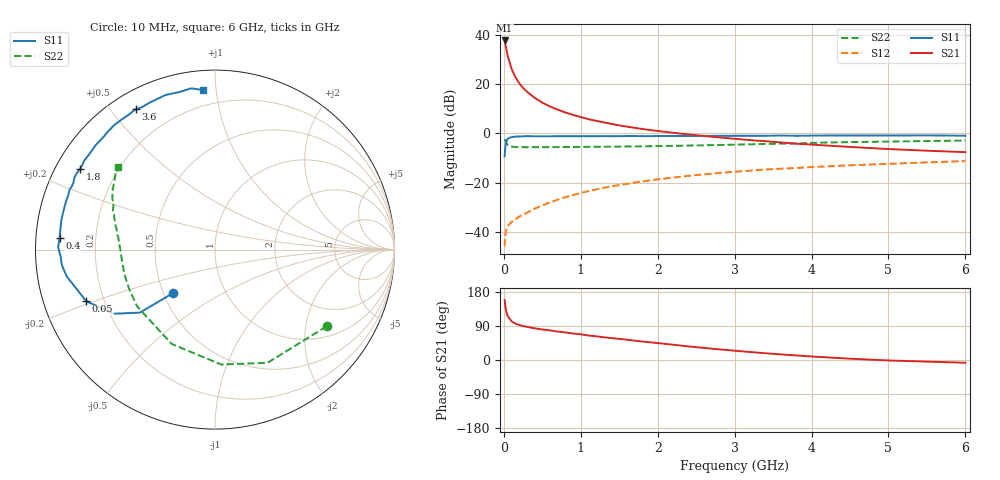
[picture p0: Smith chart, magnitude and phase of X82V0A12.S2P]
! SIEMENS Small Signal Semiconductors
! BFP136W
! Si NPN RF Bipolar Junction Transistor in SOT343
! VCE = 2 V  IC = 120 mA
! Common Emitter S-Parameters:  September  1994
# GHz  S  MA  R  50
!  f  S11  S21  S12  S22
! GHz  MAG  ANG  MAG  ANG  MAG  ANG  MAG  ANG
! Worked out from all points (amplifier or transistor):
!   40 points, 10 MHz to 6 GHz, reference 50 ohm
!   highest |S21| = 37.7 dB at 10 MHz (marker M1)
!   |S21| within 3 dB of that: start of sweep to 29.13 MHz
!   unconditionally stable (mu >= 1): 429.8 MHz to 2.936 GHz
!   at 200 MHz: K = 0.76, MSG = 27.1 dB, |S12| = -33.8 dB
!   at 1.5 GHz: K = 1.12, MAG = 10.0 dB, |S12| = -21.0 dB
!   at 6 GHz: K = 0.99, MSG = 1.8 dB, |S12| = -11.3 dB
!   S11 on the Smith chart (normalised r, x): 10 MHz: 0.56, -0.31; 50 MHz: 0.13, -0.19; 400 MHz: 0.07, +0.04; 1.8 GHz: 0.07, +0.27; 3.6 GHz: 0.07, +0.58; 6 GHz: 0.11, +0.92
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0.01  0.34 -134.1  76.86 158.7  0.0051 66.5  0.7547 -34.5
0.02  0.5462 -140.0  64.77 141.4  0.0086 54.6  0.6954 -65.1
0.03  0.6687 -147.7  53.52 129.6  0.0108 47.6  0.6412 -86.9
0.05  0.7729 -158.2  37.42 115.9  0.0131 37.9  0.5786 -114.6
0.1  0.8386 -169.6  20.41 102.1  0.0158 37.3  0.5372 -144.0
0.15  0.8581 -174.3  13.84 96.1  0.0179 42.4  0.5258 -155.7
0.2  0.8598 -177.1  10.38 92.4  0.0204 45.3  0.523 -162.0
0.25  0.8684 -179.5  8.364 89.6  0.0223 47.7  0.5227 -165.9
0.3  0.8741 179.0  6.993 87.5  0.0243 51.5  0.5212 -168.5
0.4  0.8684 175.6  5.262 83.7  0.0295 55.6  0.5223 -172.2
0.5  0.8686 173.2  4.193 80.6  0.0342 58.9  0.5226 -174.7
0.6  0.8696 171.4  3.504 78.1  0.0393 60.7  0.5236 -176.3
0.7  0.8716 169.1  3.022 75.0  0.045 62.2  0.5252 -177.6
0.9  0.871 165.6  2.365 70.0  0.0557 63.1  0.5273 180.0
1.1  0.8724 161.4  1.937 64.6  0.0668 63.1  0.5305 178.3
1.8  0.8757 149.2  1.223 48.7  0.1051 59.4  0.5428 172.7
2.2  0.8795 142.5  1.024 40.3  0.1261 56.1  0.5548 169.6
3.2  0.8921 125.7  0.728 21.1  0.1743 46.0  0.5964 160.7
3.6  0.8983 119.5  0.654 14.8  0.1909 41.9  0.6154 157.1
4.5  0.9046 107.7  0.528 3.5  0.224 33.3  0.6628 149.2
5.5  0.9083 98.5  0.443 -4.3  0.2565 25.2  0.6982 142.6
6  0.8917 94.3  0.414 -7.2  0.2724 20.8  0.7119 139.6
